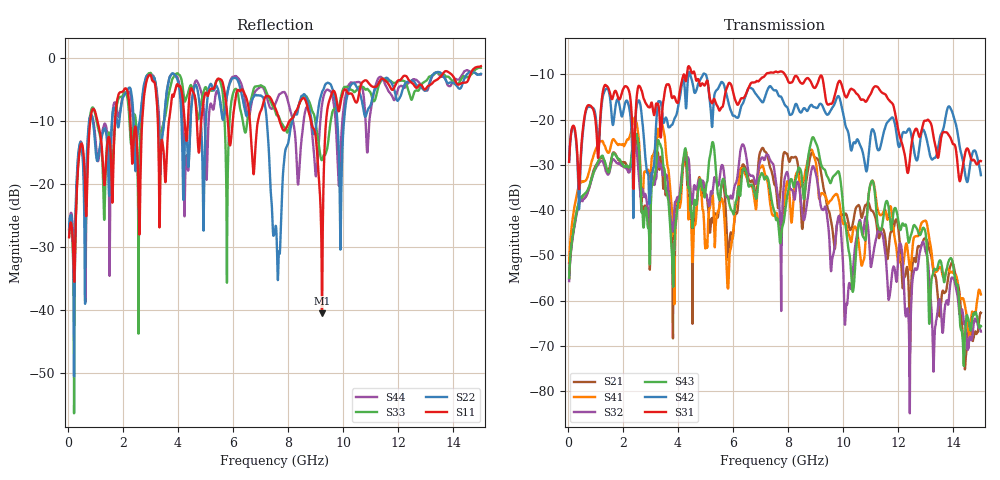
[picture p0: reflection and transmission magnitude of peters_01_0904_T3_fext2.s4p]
# MHZ S RI R 50.00
! FREQ  S11  S12  S13  S14
!  S21  S22  S23  S24
!  S31  S32  S33  S34
!  S41  S42  S43  S44
!  REAL  IMAG  REAL  IMAG  REAL  IMAG  REAL  IMAG
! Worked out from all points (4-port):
!   1496 points, 50 MHz to 15 GHz, reference 50 ohm
!   strongest paths, dB at 50 MHz, 3.79 GHz, 7.53 GHz, 11.27 GHz, 15 GHz:
!     S31: -29.3, -15.2, -9.4, -12.9, -29.1
!     S42: -29.3, -21.1, -13.5, -26.8, -32.3
!     S43: -54.9, -50.4, -41.1, -43.6, -65.6
!     S32: -55.7, -43.9, -32.4, -44.6, -66.8
!     S41: -51.6, -40.1, -40.9, -40.2, -58.6
!     S21: -55.2, -49.1, -34.4, -45.7, -62.7
!   lowest |S11| = -40.5 dB at 9.23 GHz (marker M1), VSWR 1.02, Z = 50.9 + j0.209 ohm
!   |S11| at or under -10 dB: start of sweep to 816.9 MHz; 1.08 GHz to 1.716 GHz (636.8 MHz wide, 45.5 % of centre); 8.829 GHz to 9.38 GHz (550.3 MHz wide, 6.04 % of centre)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
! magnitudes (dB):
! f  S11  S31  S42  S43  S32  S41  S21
! 50 MHz  -28.4  -29.3  -29.3  -54.9  -55.7  -51.6  -55.2
! 2.43 GHz  -11.2  -24.2  -23.9  -22.9  -24.9  -19.6  -23.6
! 3.81 GHz  -5.8  -15.2  -20.9  -53.6  -44.7  -40.8  -59.4
! 5.26 GHz  -4.9  -16.2  -20.3  -24.9  -35.9  -36.5  -42.7
! 7.65 GHz  -9.4  -9.5  -14.6  -43.3  -37.3  -42.4  -39.4
! 9.23 GHz  -40.5  -10.5  -16.7  -30.4  -39.8  -36.2  -33.0
! 15 GHz  -1.3  -29.1  -32.3  -65.6  -66.8  -58.6  -62.7
